FUNCTION_BLOCK FB72
TITLE =Get Target Position
//*****************************************************************************
//* maxon motor ag
//* R&D
//* all rights reserved
//*****************************************************************************
//* Summary:  Read target value of position
//*
//* Remarks:
//*
//* Created under: STEP7 REV5.2+SP1
//*****************************************************************************
//* History:
//* 19.05.2004 | INA   first release
//*
//*
//*****************************************************************************
//

AUTHOR:INA
FAMILY:ProPosMo
NAME:GetTarPo
VERSION:00.01


VAR_INPUT

Read : BOOL //A rising edge start the command

  NodeID : BYTE //Adress of the maxon device

END_VAR
VAR_OUTPUT
  Done : BOOL //Data valid flag is TRUE if data were available

  Err : BOOL //Error flag is TRUE if an Error has occured, see ErrNo for more details

  ErrNo : DINT //Contains detailed error information

  TargetPosition : DINT //Target Position

END_VAR
VAR
  xEdgeMerker : BOOL //Edge Merker

  xEdgeFlag : BOOL //Edge Flag

  xStep : INT
END_VAR

BEGIN

NETWORK
TITLE = Activate the service function
//

// SDO Read "Get Target Position"

       U    #Read
       FP   #xEdgeFlag                   // recognize a positiv edge of the Read signal
       =    #xEdgeMerker                 // and set the xEdgeMerker for one cycle to true

       L    #xStep
       L    0
       ==I
       U    #xEdgeMerker
       SPB  nstp                         // iStep = 1 -> fnc1

       L    #xStep                       // jump list
       SPL  List
       SPA  rdef
       SPA  fnc1
       SPA  fncE
List  :SPA  rdef

rdef  :NOP  0
       R    #Done                        // reset Done
       R    #Err                         // reset Error
       L    0
       T    #xStep                       // iStep = 0
       SPA  end

fnc1  :NOP  0
       CALL FC1
         NodeID:=#NodeID
         Index:=DW#16#0000607A
         SubIndex:=DW#16#00000000
         RET_VAL:=#Done
         Err:=#Err
         ErrNo:=#ErrNo

       L    DB219.DBD10
       T    #TargetPosition

       L    1
       U    #Err
       SPB  fncE

       SPA  nstp                         // iStep = 1 -> fnc2

fncE  :NOP  0
       L    0
       T    #xStep
       SPA  end

nstp  :NOP  0
       L    #xStep
       INC            1
       T    #xStep

end   :NOP  0
END_FUNCTION_BLOCK
